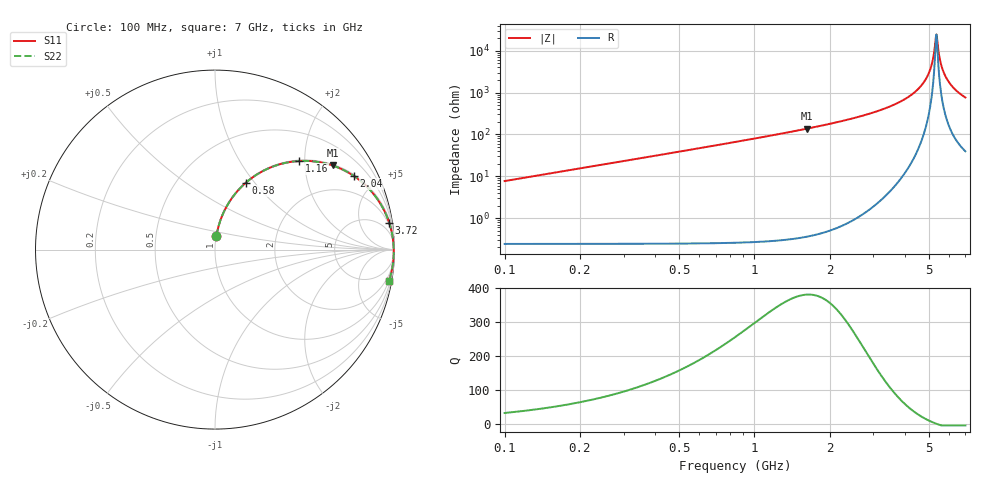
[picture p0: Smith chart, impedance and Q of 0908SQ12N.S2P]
! Coilcraft 0908SQ-12N Air Core Inductor
! 06 March 2008
# MHZ S MA R 50
!Freq  MagS11  AngS11  MagS21  AngS21  MagS12  AngS12  MagS22  AngS22
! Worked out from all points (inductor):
!   346 points, 100 MHz to 7 GHz, reference 50 ohm
!   read as one part in series: L = 12.2 nH near 120 MHz
!   highest Q = 382 at 1.62 GHz (marker M1), where L = 13.4 nH
!   self-resonance near 5.34 GHz
!   S11 on the Smith chart (normalised r, x): 100 MHz: 1.00, +0.15; 580 MHz: 1.01, +0.90; 1.16 GHz: 1.02, +1.87; 2.04 GHz: 1.06, +3.74; 3.72 GHz: 2, +13; 7 GHz: 1, -11
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100  0.07607 83.8  0.9947 -4.4  0.9947 -4.4  0.07608 83.8
180  0.1361 81.1  0.9883 -7.9  0.9883 -7.9  0.1361 81.1
280  0.2093 77.2  0.9755 -12.2  0.9755 -12.2  0.2093 77.2
580  0.4084 65.4  0.9106 -24.3  0.9106 -24.3  0.4084 65.4
1160  0.6801 46.5  0.7311 -43.3  0.7311 -43.3  0.6801 46.5
1260  0.7129 43.9  0.6992 -46.0  0.6992 -46.0  0.7129 43.9
1620  0.8053 35.6  0.5907 -54.3  0.5907 -54.3  0.8053 35.6
2040  0.8759 27.9  0.48 -61.9  0.48 -61.9  0.8759 27.9
2400  0.9157 22.6  0.3986 -67.2  0.3986 -67.2  0.9157 22.6
3560  0.9777 10.2  0.2002 -79.3  0.2002 -79.3  0.9778 10.2
3720  0.9818 8.8  0.1784 -80.5  0.1784 -80.5  0.9818 8.8
4700  0.9948 1.8  0.06367 -85.3  0.06367 -85.3  0.9948 1.8
4940  0.9957 0.3  0.03955 -84.6  0.03955 -84.6  0.9957 0.3
5120  0.996 -0.7  0.02236 -81.1  0.02236 -81.1  0.996 -0.7
5240  0.996 -1.4  0.01152 -71.7  0.01152 -71.7  0.9961 -1.4
5340  0.9959 -2.0  0.004377 -24.8  0.004377 -24.8  0.996 -2.0
5360  0.9959 -2.1  0.004064 -0.6  0.004064 -0.6  0.996 -2.1
5480  0.9957 -2.8  0.0116 65.8  0.0116 65.8  0.9957 -2.8
5560  0.9955 -3.2  0.01832 73.1  0.01832 73.1  0.9955 -3.2
5860  0.9943 -4.8  0.04339 78.9  0.04339 78.9  0.9943 -4.8
6320  0.9913 -7.1  0.07968 79.0  0.07968 79.0  0.9913 -7.1
7000  0.985 -10.2  0.1287 76.9  0.1287 76.9  0.9851 -10.2
